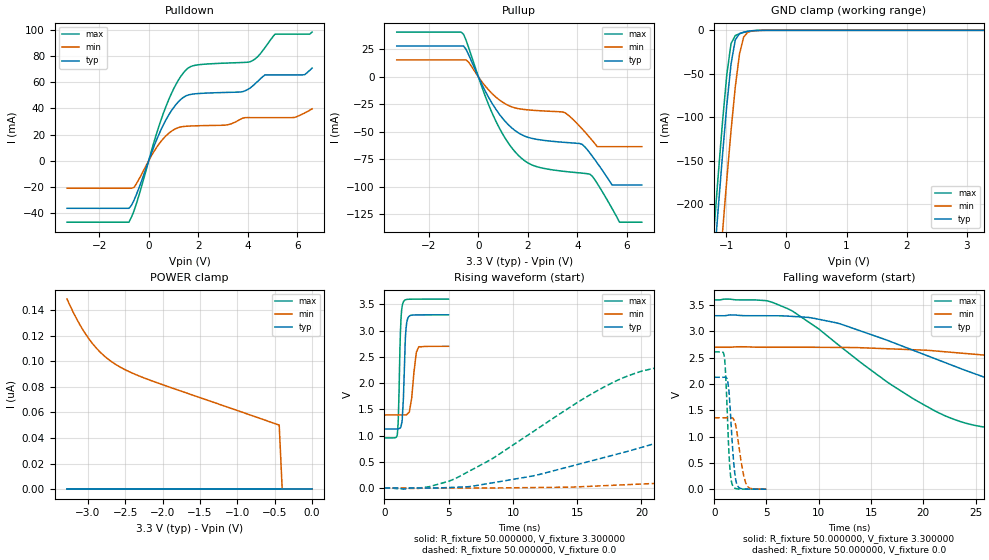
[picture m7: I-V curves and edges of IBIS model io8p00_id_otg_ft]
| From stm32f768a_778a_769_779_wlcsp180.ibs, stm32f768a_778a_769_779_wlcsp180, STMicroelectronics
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|   Model io8p00_id_otg_ft
[Model]  io8p00_id_otg_ft
Model_type I/O
Polarity   Non-Inverting
Enable   Active-Low
Vinl =   0.990000V
Vinh =   2.310000V
Vmeas =  1.650000V
Cref =   50.000000pF
Rref =   100.000000M
Vref =   0.0V
C_comp   2.282200pF   2.214200pF   2.357400pF
[Temperature Range]   25.000000   0.125000k   -40.000000
[Pullup Reference]   3.300000V   2.700000V   3.600000V
[Pulldown Reference]   0.0V   0.0V   0.0V
[POWER Clamp Reference]   3.300000V   2.700000V   3.600000V
[GND Clamp Reference]   0.0V   0.0V   0.0V
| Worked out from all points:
|   slope of the pulldown table from 0 to 0.495 V, typ, clamps not added: 20.9 ohm
|   slope of the pullup table from 0 to 0.495 V, typ, clamps not added: 22.6 ohm
|   GND clamp passes 1 mA (typ) near -0.62 V on its own axis
|   rising waveform, R_fixture 50.000000, V_fixture 3.300000: 20-80 % time 191ps typ, 330ps min, 165ps max; typ from 1.12 V to 3.3 V
|   rising waveform, R_fixture 50.000000, V_fixture 0.0: 20-80 % time 19.7ns typ, 51ns min, 10.3ns max; typ from 0 V to 2.13 V
|   falling waveform, R_fixture 50.000000, V_fixture 3.300000: 20-80 % time 18.6ns typ, 38.5ns min, 11.3ns max; typ from 3.3 V to 1.12 V
|   falling waveform, R_fixture 50.000000, V_fixture 0.0: 20-80 % time 435ps typ, 634ps min, 344ps max; typ from 2.13 V to 0 V
[Pulldown]
|Voltage   I(typ)   I(min)   I(max)
-3.3V     -36.46mA   -21.09mA   -47.09mA
-800mV    -36.46mA   -21.09mA   -47.09mA
-600mV    -30.5mA    -20.54mA   -38.68mA
700mV     31.4mA     19.11mA    41.71mA
1.2V      45.15mA    25.37mA    61.75mA
1.6V      50.35mA    26.5mA     71.06mA
3.1V      52.28mA    27.26mA    74.76mA
4.1V      55.71mA    33mA       75.81mA
4.7V      65.72mA    33mA       86.7mA
5.1V      65.72mA    33mA       96.91mA
6.3V      65.88mA    36.51mA    96.91mA
6.6V      70.94mA    39.72mA    98.51mA
[Pullup]
|Voltage   I(typ)   I(min)   I(max)
-3.3V     28.04mA    15.43mA    40.7mA
-700mV    28.04mA    15.43mA    40.7mA
-400mV    20.31mA    13.47mA    26.93mA
600mV     -25.77mA   -16.23mA   -35.14mA
1.6V      -50.64mA   -28.81mA   -70.96mA
3.5V      -59.53mA   -32.65mA   -85.92mA
4.2V      -61.43mA   -47.49mA   -87.46mA
4.5V      -69.06mA   -55.12mA   -88.38mA
4.8V      -78.22mA   -63.4mA    -96.84mA
5.4V      -98.2mA    -63.4mA    -119.6mA
5.7V      -98.2mA    -63.4mA    -132mA
6.6V      -98.2mA    -63.4mA    -132mA
[GND_clamp]
|Voltage   I(typ)   I(min)   I(max)
-3.3V     -2.319A    -2.398A    -2.292A
-1.2V     -265.5mA   -356.1mA   -227.2mA
-1.13V    -202.7mA   -292.9mA   -164.1mA
-1.06V    -142.2mA   -231.2mA   -104.1mA
-990mV    -85.98mA   -171.6mA   -50.73mA
-920mV    -38.81mA   -115.5mA   -15.3mA
-850mV    -11.1mA    -65.61mA   -6.021mA
-780mV    -3.796mA   -27.43mA   -3.892mA
-710mV    -2.096mA   -7.699mA   -2.393mA
-640mV    -1.154mA   -2.125mA   -1.227mA
-570mV    -528.1uA   -803.6uA   -480.7uA
3.28V     0A         0A         0A
[POWER_clamp]
|Voltage   I(typ)   I(min)   I(max)
-3.28V    0A         148.5nA    0A
-3.2V     0A         138.6nA    0A
-3.12V    0A         129.7nA    0A
-3.04V    0A         122nA      0A
-2.96V    0A         115.3nA    0A
-2.8V     0A         105.1nA    0A
-2.6V     0A         96.44nA    0A
-2.4V     0A         90.52nA    0A
-2.16V    0A         84.97nA    0A
-440mV    0A         50.04nA    0A
-400mV    0A         0A         0A
0V        0A         0A         0A
[Ramp]
| variable   typ   min   max
dV/dt_r  1.27740/19.68819n   0.81540/50.98348n   1.56732/10.32904n
dV/dt_f  1.30710/18.56865n   0.78486/38.55583n   1.58789/11.32467n
R_load = 50.000000
[Rising Waveform]
R_fixture= 50.000000
V_fixture= 3.300000
V_fixture_min= 2.700000
V_fixture_max= 3.600000
|time   V(typ)   V(min)   V(max)
0s        1.124V     1.392V     953.5mV
1.001ns   1.126V     1.392V     1.018V
1.071ns   1.128V     1.392V     1.288V
1.251ns   1.149V     1.392V     3.031V
1.461ns   1.659V     1.391V     3.54V
1.632ns   2.879V     1.394V     3.586V
1.862ns   3.257V     1.43V      3.596V
2.482ns   3.298V     2.587V     3.599V
2.663ns   3.299V     2.689V     3.599V
4.985ns   3.3V       2.7V       3.6V
[Rising Waveform]
R_fixture= 50.000000
V_fixture= 0.0
V_fixture_min= 0.0
V_fixture_max= 0.0
|time   V(typ)   V(min)   V(max)
0s        4.932nV    245.7nV    3.133nV
5.506ns   13.81mV    -140.2uV   177.7mV
11.51ns   227.5mV    8.258mV    1.064V
19.02ns   703.8mV    64.87mV    2.142V
27.53ns   1.299V     163.4mV    2.488V
38.54ns   1.854V     360.2mV    2.577V
57.56ns   2.068V     710.1mV    2.609V
89.09ns   2.119V     1.139V     2.612V
117.6ns   2.128V     1.298V     2.612V
249.2ns   2.129V     1.359V     2.612V
[Falling Waveform]
R_fixture= 50.000000
V_fixture= 3.300000
V_fixture_min= 2.700000
V_fixture_max= 3.600000
|time   V(typ)   V(min)   V(max)
0s        3.3V       2.7V       3.6V
5.506ns   3.299V     2.7V       3.559V
12.01ns   3.148V     2.696V     2.724V
22.02ns   2.413V     2.615V     1.401V
31.03ns   1.761V     2.445V     1.08V
38.54ns   1.414V     2.264V     1.022V
46.05ns   1.28V      2.078V     999mV
62.56ns   1.186V     1.739V     970.3mV
87.09ns   1.145V     1.524V     957mV
249.2ns   1.124V     1.392V     953.5mV
[Falling Waveform]
R_fixture= 50.000000
V_fixture= 0.0
V_fixture_min= 0.0
V_fixture_max= 0.0
|time   V(typ)   V(min)   V(max)
0s        2.129V     1.359V     2.612V
981ps     2.13V      1.359V     2.507V
1.151ns   2.12V      1.358V     1.948V
1.411ns   1.87V      1.359V     689.3mV
1.542ns   1.49V      1.361V     300.5mV
1.742ns   834.4mV    1.354V     80.25mV
2.152ns   102.7mV    1.12V      8.45mV
2.833ns   4.224mV    246.8mV    456.5uV
3.123ns   1.431mV    74.07mV    294.2uV
4.985ns   4.932nV    245.7nV    3.133nV
